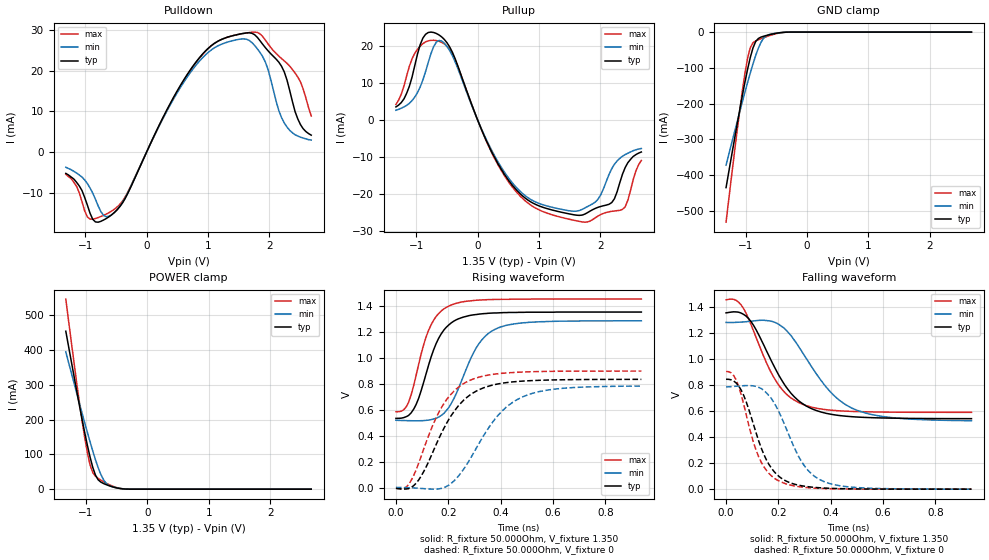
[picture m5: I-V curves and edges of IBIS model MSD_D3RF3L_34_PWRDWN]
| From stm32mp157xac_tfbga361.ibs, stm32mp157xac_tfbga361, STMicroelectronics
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[Model] MSD_D3RF3L_34_PWRDWN
Model_type   I/O
C_comp 2.572pF   2.485pF   2.698pF
Vinh = 810.000mV
Vinl = 540.000mV
Vmeas = 675.000mV
Vref = 675.000mV
[Model Spec]
Vinh   810.000mV   777.000mV   860.000mV
Vinl   540.000mV   507.000mV   590.000mV
Vmeas   675.000mV   642.000mV   725.000mV
Vref   675.000mV   642.000mV   725.000mV
[Temperature Range]   25.000   125.000   -40.000
[Voltage Range]   1.350V   1.283V   1.450V
[GND Clamp Reference]   0.00V   0.00V   0.00V
[Pulldown Reference]   0.00V   0.00V   0.00V
[POWER Clamp Reference]   1.350V   1.283V   1.450V
[Pullup Reference]   1.350V   1.283V   1.450V
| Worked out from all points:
|   slope of the pulldown table from 0 to 0.203 V, typ, clamps not added: 31 ohm
|   slope of the pullup table from 0 to 0.203 V, typ, clamps not added: 26.2 ohm
|   GND clamp passes 1 mA (typ) near -0.40 V on its own axis
|   POWER clamp passes 1 mA (typ) near -0.41 V on its own axis
|   rising waveform, R_fixture 50.000Ohm, V_fixture 1.350: 20-80 % time 86.2ps typ, 108ps min, 77.1ps max; typ from 0.532 V to 1.35 V
|   rising waveform, R_fixture 50.000Ohm, V_fixture 0: 20-80 % time 139ps typ, 162ps min, 125ps max; typ from -0.006 V to 0.832 V
|   falling waveform, R_fixture 50.000Ohm, V_fixture 1.350: 20-80 % time 140ps typ, 171ps min, 124ps max; typ from 1.36 V to 0.542 V
|   falling waveform, R_fixture 50.000Ohm, V_fixture 0: 20-80 % time 94.9ps typ, 115ps min, 83.9ps max; typ from 0.846 V to 0 V
[GND Clamp]
-1.318V   -435mA     -372.2mA   -531.7mA
-1.142V   -262.4mA   -254.2mA   -282.5mA
-1.055V   -179.8mA   -196.6mA   -167.2mA
-1.011V   -140.5mA   -168.4mA   -116mA
-966.7mV  -103.7mA   -140.9mA   -72.98mA
-922.7mV  -70.73mA   -114.2mA   -43.23mA
-878.8mV  -44.02mA   -88.84mA   -29.72mA
-790.9mV  -17.74mA   -44.62mA   -21.37mA
-703mV    -11.46mA   -16.55mA   -15.5mA
-527.3mV  -4.197mA   -3.553mA   -5.598mA
-263.6mV  -40.6uA    -78.9uA    -28.72uA
2.68V     28.25nA    782nA      4.355nA
[Power Clamp]
-1.33V    454.4mA    394.7mA    546.8mA
-1.111V   243.5mA    248.7mA    252.9mA
-1.023V   163.7mA    191.5mA    149.8mA
-978.8mV  126.5mA    163.6mA    105.2mA
-934.9mV  92.34mA    136.2mA    69.61mA
-890.9mV  62.88mA    109.8mA    47.89mA
-847mV    40.47mA    84.8mA     37.29mA
-803mV    27.03mA    61.92mA    31.1mA
-715.1mV  16.21mA    27.03mA    21.42mA
-671.2mV  12.92mA    16.88mA    17.18mA
-407.6mV  989.1uA    1.283mA    1.2mA
2.668V    -48.24nA   -903.5nA   -4.583nA
[Pulldown]
-1.318V   -5.3mA     -3.8mA     -5.5mA
-966.7mV  -13.1mA    -7.8mA     -16.01mA
-834.9mV  -17.24mA   -11.67mA   -16.39mA
-571.2mV  -15.49mA   -15.46mA   -14.56mA
-351.5mV  -11.48mA   -11.33mA   -11.1mA
747mV     20.95mA    20.23mA    20.78mA
1.098V    26.62mA    25.53mA    26.63mA
1.582V    29.15mA    27.77mA    29.12mA
1.933V    25.62mA    22.07mA    27.48mA
2.197V    21.03mA    8.4mA      22.94mA
2.461V    8.1mA      3.9mA      18.4mA
2.68V     4.1mA      2.9mA      8.8mA
[Pullup]
-1.33V    3.5mA      2.605mA    4.152mA
-1.023V   14.7mA     6.177mA    18.04mA
-890.9mV  22.15mA    10.8mA     20.65mA
-715.1mV  23.66mA    19.86mA    21.55mA
-451.5mV  19.67mA    18.67mA    18.98mA
251.5mV   -9.374mA   -8.925mA   -9.602mA
866.7mV   -22.22mA   -21.57mA   -23.09mA
1.702V    -25.79mA   -24.26mA   -27.63mA
1.965V    -23.66mA   -21.43mA   -26.01mA
2.185V    -22.41mA   -13.25mA   -24.77mA
2.361V    -14.7mA    -9.838mA   -24.24mA
2.668V    -8.7mA     -7.748mA   -10.98mA
[Ramp]
R_load=50.000Ohm
dV/dt_r   492.120mV/113.000ps  462.689mV/135.000ps  526.590mV/101.500ps
dV/dt_f   492.120mV/117.500ps  462.689mV/144.000ps  526.590mV/104.000ps
[Rising waveform]
R_fixture=50.000Ohm
V_fixture=1.350
V_fixture_min=1.283
V_fixture_max=1.450
0s        532.1mV    517.5mV    583mV
39ps      544.7mV    515mV      619.6mV
68ps      603.6mV    513.7mV    785.6mV
125ps     942.9mV    519mV      1.211V
163ps     1.147V     541.8mV    1.338V
202ps     1.251V     615.1mV    1.396V
307ps     1.331V     1.075V     1.441V
384ps     1.343V     1.222V     1.447V
508ps     1.349V     1.271V     1.449V
938ps     1.35V      1.283V     1.45V
[Rising waveform]
R_fixture=50.000Ohm
V_fixture=0
0s        -6.207mV   775.4uV    -5.773mV
48ps      -8.52mV    -1.234mV   22.37mV
87ps      58.48mV    -5.313mV   187.6mV
173ps     414.4mV    -6.698mV   611.6mV
221ps     581.4mV    49.26mV    740.1mV
269ps     690.1mV    172mV      811.4mV
384ps     794.6mV    540.5mV    874.3mV
480ps     818.3mV    693.9mV    888.2mV
614ps     828.4mV    758.9mV    894.4mV
938ps     832.3mV    780.8mV    896mV
[Falling waveform]
R_fixture=50.000Ohm
V_fixture=1.350
V_fixture_min=1.283
V_fixture_max=1.450
0s        1.356V     1.282V     1.456V
48ps      1.361V     1.284V     1.438V
87ps      1.31V      1.29V      1.307V
183ps     947.3mV    1.285V     858.1mV
221ps     811.7mV    1.24V      751.2mV
278ps     678.7mV    1.095V     665.7mV
393ps     579.1mV    760.8mV    609mV
499ps     555mV      607.4mV    596.9mV
633ps     546.2mV    550.2mV    592.2mV
938ps     542.3mV    526.4mV    590.9mV
[Falling waveform]
R_fixture=50.000Ohm
V_fixture=0
0s        845.5mV    785.9mV    905mV
29ps      832.2mV    790mV      874.7mV
58ps      761.3mV    794.6mV    725.6mV
106ps     490.4mV    793.8mV    351.9mV
135ps     314mV      772.9mV    205.2mV
202ps     98.51mV    595.1mV    63.08mV
288ps     26.51mV    213.6mV    16.69mV
374ps     8.78mV     58.4mV     4.638mV
518ps     1.484mV    10.34mV    665.5uV
938ps     31.09uV    167.6uV    -8.164uV
